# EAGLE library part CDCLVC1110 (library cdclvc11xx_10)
CDCLVC1110 3.3V and 2.5V LVCMOS High-Performance Clock Buffer - 1:10 Fan-out Source: http://www.ti.com/lit/ds/symlink/cdclvc1110.pdf
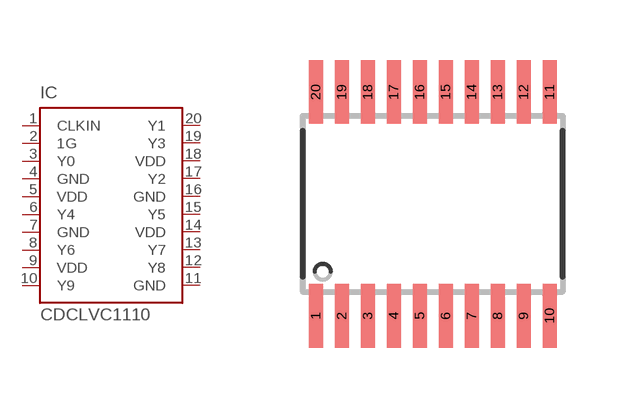
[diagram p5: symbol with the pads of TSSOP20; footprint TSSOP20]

Designator prefix IC

## CDCLVC1110PW (MF: Texas Instruments; MPN: CDCLVC1110; OC_FARNELL: unknown; OC_NEWARK: 79R7916)  [TSSOP20]
1  CLKIN  in
2  1G  in
3  Y0  out
4  GND  pwr
5  VDD  pwr
6  Y4  out
7  GND  pwr
8  Y6  out
9  VDD  pwr
10  Y9  out
11  GND  pwr
12  Y8  out
13  Y7  out
14  VDD  pwr
15  Y5  out
16  GND  pwr
17  Y2  out
18  VDD  pwr
19  Y3  out
20  Y1  out

## Footprint TSSOP20 (pad centres in mm)
TSSOP-20 Plastic Thin Srink Small Outline (PW) Source: http://www.ti.com/lit/ds/symlink/cdclvc1110.pdf
smd 0.35 x 1.6: 1 -2.925,-2.8; 2 -2.275,-2.8; 3 -1.625,-2.8; 4 -0.975,-2.8; 5 -0.325,-2.8; 6 0.325,-2.8; 7 0.975,-2.8; 8 1.625,-2.8; 9 2.275,-2.8; 10 2.925,-2.8; 11 2.925,2.8; 12 2.275,2.8; 13 1.625,2.8; 14 0.975,2.8; 15 0.325,2.8; 16 -0.325,2.8; 17 -0.975,2.8; 18 -1.625,2.8; 19 -2.275,2.8; 20 -2.925,2.8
